TYPE STR_HEATER_LINE_CUS_IN :
STRUCT
	SBrkAlarm_EN	:	USINT	;
	Temp_Hi_Alarm_Inhibit	:	USINT	;
	Inhibit_Buffer	:	REAL	;
	RateUp	:	REAL	;
	RateDown	:	REAL	;
	PID_P	:	REAL	;
	PID_I	:	REAL	;
	PID_D	:	REAL	;
	AutotuneActivate	:	USINT	;
	Autotune_Status	:	USINT	;
	Autotune_PID_P:REAL;
	Autotune_PID_I:REAL;
	Autotune_PID_D:REAL;
END_STRUCT
END_TYPE
